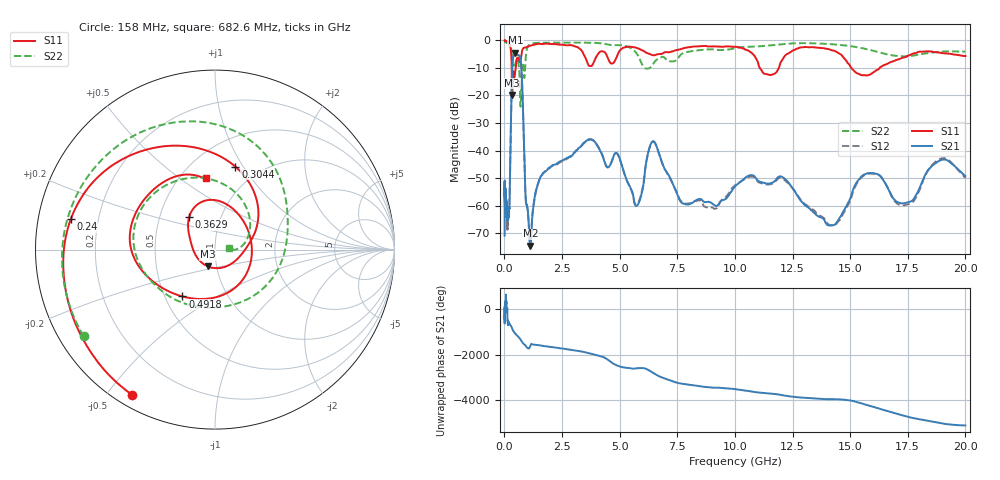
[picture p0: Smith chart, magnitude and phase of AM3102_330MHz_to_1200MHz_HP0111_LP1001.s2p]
! Date/Time: Tue, Sep 11, 2018 5:16 PM
! Network Analyzer: Agilent Technologies E8362B Rev: A.07.50.63
! Sweep from 0.010 to 20.000 GHz, 1601 Points, Sweep Type: LOG
! Power Supply: 4.949 V, 0.001 A
# Hz S DB R 50
!freq MagS11 AngS11 MagS21 AngS21 MagS12 AngS12 MagS22 AngS22
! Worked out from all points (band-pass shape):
!   1601 points, 10 MHz to 20 GHz, reference 50 ohm
!   highest |S21| = -4.38 dB at 475.7 MHz (marker M1); lowest = -74.6 dB at 1.129 GHz (marker M2)
!   |S21| within 3 dB of the highest: 360.9 MHz to 709.2 MHz (348.3 MHz wide, 65.1 % of centre)
!   lowest |S11| = -19.8 dB at 341.1 MHz (marker M3), VSWR 1.23, Z = 45.4 - j8.57 ohm
!   |S11| at or under -10 dB: 317.4 MHz to 491.2 MHz (173.8 MHz wide, 43 % of centre); 11.09 GHz to 11.91 GHz (823.1 MHz wide, 7.16 % of centre); 15.04 GHz to 16.28 GHz (1.234 GHz wide, 7.88 % of centre)
!   |S22| runs from -24.1 to -0.3 dB; largest |S21 - S12| = 0.011
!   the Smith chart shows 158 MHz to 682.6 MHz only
!   S11 on the Smith chart (normalised r, x): 158 MHz: 0.05, -0.58; 240 MHz: 0.10, +0.10; 304.4 MHz: 0.77, +0.92; 362.9 MHz: 0.71, +0.27; 491.8 MHz: 0.61, -0.36; 682.6 MHz: 0.67, +0.63
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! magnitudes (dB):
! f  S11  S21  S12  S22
! 10 MHz  0.0  -71.0  -55.4  -0.3
! 10.79 MHz  0.0  -51.5  -53.1  -0.3
! 35.55 MHz  0.0  -57.4  -58.5  -0.5
! 126.4 MHz  -0.4  -64.8  -66.4  -1.0
! 158 MHz  -0.6  -63.6  -65.5  -1.1
! 240 MHz  -1.7  -51.9  -52.1  -1.8
! 304.4 MHz  -6.4  -21.1  -21.2  -3.4
! 341.1 MHz  -19.8  -9.8  -9.9  -6.6
! 362.9 MHz  -12.7  -7.2  -7.3  -8.2
! 447.2 MHz  -12.9  -4.4  -4.5  -9.3
! 475.7 MHz  -11.2  -4.4  -4.4  -8.5
! 491.8 MHz  -10.0  -4.4  -4.5  -7.9
! 682.6 MHz  -7.9  -6.0  -6.1  -21.8
! 1.129 GHz  -1.9  -74.6  -74.8  -1.3
! 1.59 GHz  -1.3  -49.3  -49.4  -0.8
! 3.757 GHz  -9.3  -36.0  -35.9  -0.8
! 5.652 GHz  -2.5  -59.5  -59.0  -3.9
! 6.457 GHz  -5.4  -36.6  -36.8  -8.5
! 7.845 GHz  -2.7  -59.5  -59.3  -4.4
! 11.92 GHz  -9.9  -49.5  -50.0  -1.5
! 14.01 GHz  -3.1  -67.1  -66.4  -1.2
! 20 GHz  -5.7  -49.3  -50.0  -4.1
